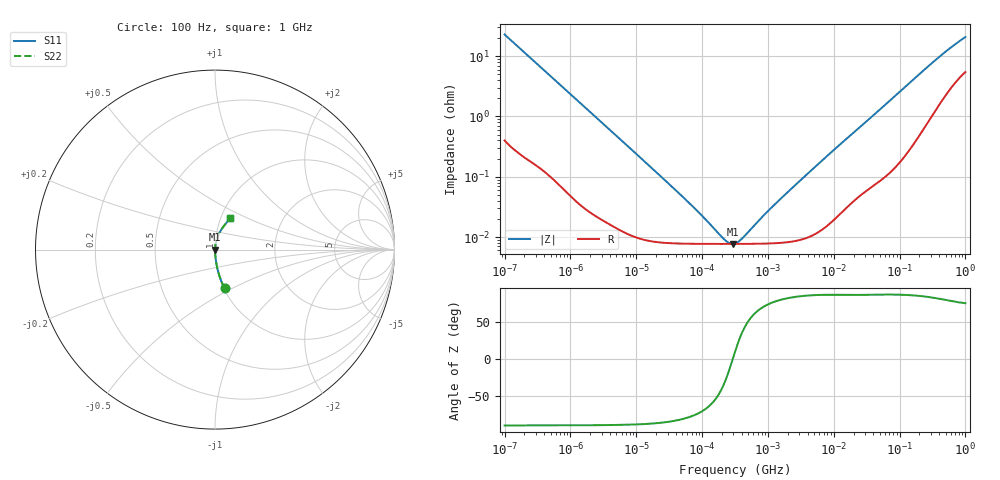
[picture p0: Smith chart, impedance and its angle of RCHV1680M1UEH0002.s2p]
! RCHV1680M1UEH0002  S-PARAMETER MODEL  (AEC-Q200 qualified)
! Model Generated by ELNA Corporation (http://www.ty-top.com)
! Version 1.0
! ELNA Control No. 240229
! Copyright (c) 2024 ELNA CO.,LTD. All Rights Reserved.
! Products Name : CONDUCTIVE POLYMER HYBRID ALUMINUM ELECTROLYTIC CAPACITORS
! Characteristics :
!  Capacitance  :  68uF  ,  Rated voltage  :  50V
!  Operating Temp. Range  :  -55 to +105 degC  ,  Endurance  :  5000hr at 105 degC
!  Dimension D  :  8mm  ,  Dimension L  :  10mm
! Frequency Range : 100Hz - 1GHz
! External Node Assignments :
!  1  o---| |---o  2
# MHz S RI R 50
!Freq[MHz].  S11 Real  S11 Imag  S21 Real  S21 Imag  S12 Real  S12 Imag  S22 Real  S22 Imag
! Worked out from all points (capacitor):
!   401 points, 100 Hz to 1 GHz, reference 50 ohm
!   read as one part in series: C = 69.5 uF near 108 Hz
!   lowest |Z| = 7.71 mohm at 291.7 kHz (marker M1)
!   series resonance near 292.1 kHz, so ESL is about 4.3 nH
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0.0001  0.0532 -0.2158  0.9468 0.2158  0.9468 0.2158  0.0532 -0.2158
0.000113  0.0426 -0.1935  0.9574 0.1935  0.9574 0.1935  0.0426 -0.1935
0.000183  0.0176 -0.1229  0.9824 0.1229  0.9824 0.1229  0.0176 -0.1229
0.000309  0.00703 -0.0741  0.993 0.0741  0.993 0.0741  0.00703 -0.0741
0.000613  0.00225 -0.0379  0.9978 0.0379  0.9978 0.0379  0.00225 -0.0379
0.001488  0.000575 -0.0158  0.9994 0.0158  0.9994 0.0158  0.000575 -0.0158
0.022131  8.3e-05 -0.00108  0.9999 0.00108  0.9999 0.00108  8.3e-05 -0.00108
0.080353  7.75e-05 -0.000277  0.9999 0.000277  0.9999 0.000277  7.75e-05 -0.000277
0.187284  7.71e-05 -7.56e-05  0.9999 7.56e-05  0.9999 7.56e-05  7.71e-05 -7.56e-05
0.211349  7.71e-05 -5.42e-05  0.9999 5.42e-05  0.9999 5.42e-05  7.71e-05 -5.42e-05
0.291743  7.71e-05 -1.71e-07  0.9999 1.71e-07  0.9999 1.71e-07  7.71e-05 -1.71e-07
0.316228  7.71e-05 1.31e-05  0.9999 -1.31e-05  0.9999 -1.31e-05  7.71e-05 1.31e-05
0.402717  7.72e-05 5.39e-05  0.9999 -5.39e-05  0.9999 -5.39e-05  7.72e-05 5.39e-05
0.454465  7.73e-05 7.52e-05  0.9999 -7.52e-05  0.9999 -7.52e-05  7.73e-05 7.52e-05
0.767361  7.78e-05 0.000185  0.9999 -0.000185  0.9999 -0.000185  7.78e-05 0.000185
1.148154  7.89e-05 0.000303  0.9999 -0.000303  0.9999 -0.000303  7.89e-05 0.000303
4.704354  0.000108 0.00132  0.9999 -0.00132  0.9999 -0.00132  0.000108 0.00132
69.9842  0.00147 0.0179  0.9985 -0.0179  0.9985 -0.0179  0.00147 0.0179
176.8072  0.00589 0.0441  0.9941 -0.0441  0.9941 -0.0441  0.00589 0.0441
380.1894  0.0221 0.0884  0.9779 -0.0884  0.9779 -0.0884  0.0221 0.0884
668.3439  0.0523 0.1356  0.9477 -0.1356  0.9477 -0.1356  0.0523 0.1356
1000  0.0849 0.1741  0.9151 -0.1741  0.9151 -0.1741  0.0849 0.1741
